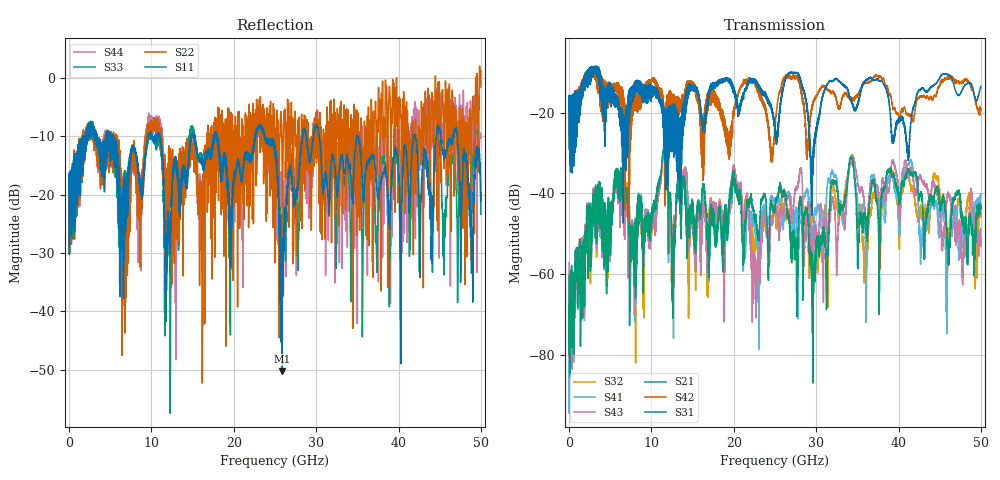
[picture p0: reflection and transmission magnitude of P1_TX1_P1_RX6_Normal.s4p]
!Keysight Technologies,N5225B,MY57041031,A.13.20.10
!Date: Friday, May 31, 2019 11:22:11
!Correction: S11(Full 4 Port(1,2,3,4))
!S12(Full 4 Port(1,2,3,4))
!S13(Full 4 Port(1,2,3,4))
!S14(Full 4 Port(1,2,3,4))
!S21(Full 4 Port(1,2,3,4))
!S22(Full 4 Port(1,2,3,4))
!S23(Full 4 Port(1,2,3,4))
!S24(Full 4 Port(1,2,3,4))
!S31(Full 4 Port(1,2,3,4))
!S32(Full 4 Port(1,2,3,4))
!S33(Full 4 Port(1,2,3,4))
!S34(Full 4 Port(1,2,3,4))
!S41(Full 4 Port(1,2,3,4))
!S42(Full 4 Port(1,2,3,4))
!S43(Full 4 Port(1,2,3,4))
!S44(Full 4 Port(1,2,3,4))
!S4P File: Measurements: <S11,S12,S13,S14>,
!<S21,S22,S23,S24>,
!<S31,S32,S33,S34>,
!<S41,S42,S43,S44>:
# Hz S  dB  R 50.0
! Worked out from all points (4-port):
!   5000 points, 10 MHz to 50 GHz, reference 50 ohm
!   strongest paths, dB at 10 MHz, 12.51 GHz, 25.01 GHz, 37.51 GHz, 50 GHz:
!     S31: -19.4, -29.3, -24.5, -11.8, -13.5
!     S42: -19.4, -15.7, -23.0, -11.0, -19.1
!     S21: -60.5, -54.0, -44.0, -45.0, -43.3
!     S43: -57.2, -49.9, -43.5, -39.4, -51.4
!     S41: -59.5, -54.8, -42.5, -42.0, -40.3
!     S32: -72.7, -53.1, -43.6, -42.8, -45.9
!   lowest |S11| = -50.2 dB at 25.83 GHz (marker M1), VSWR 1.01, Z = 49.9 + j0.3 ohm
!   |S11| at or under -10 dB: 18.01 GHz to 22.61 GHz (4.596 GHz wide, 22.6 % of centre); 30.38 GHz to 34.94 GHz (4.562 GHz wide, 14 % of centre); 34.98 GHz to 41.81 GHz (6.838 GHz wide, 17.8 % of centre)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
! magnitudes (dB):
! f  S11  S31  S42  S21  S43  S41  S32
! 10 MHz  -19.9  -19.4  -19.4  -60.5  -57.2  -59.5  -72.7
! 5.75 GHz  -12.7  -17.0  -14.8  -33.8  -36.2  -34.4  -35.5
! 23.26 GHz  -8.2  -14.6  -16.1  -43.3  -53.0  -48.6  -49.3
! 25.83 GHz  -50.2  -16.0  -12.9  -39.8  -44.6  -46.9  -41.1
! 28.56 GHz  -8.6  -15.0  -18.8  -45.4  -56.0  -41.0  -45.3
! 34.39 GHz  -19.8  -17.6  -16.6  -31.7  -30.9  -32.3  -31.0
! 50 GHz  -19.7  -13.5  -19.1  -43.3  -51.4  -40.3  -45.9
